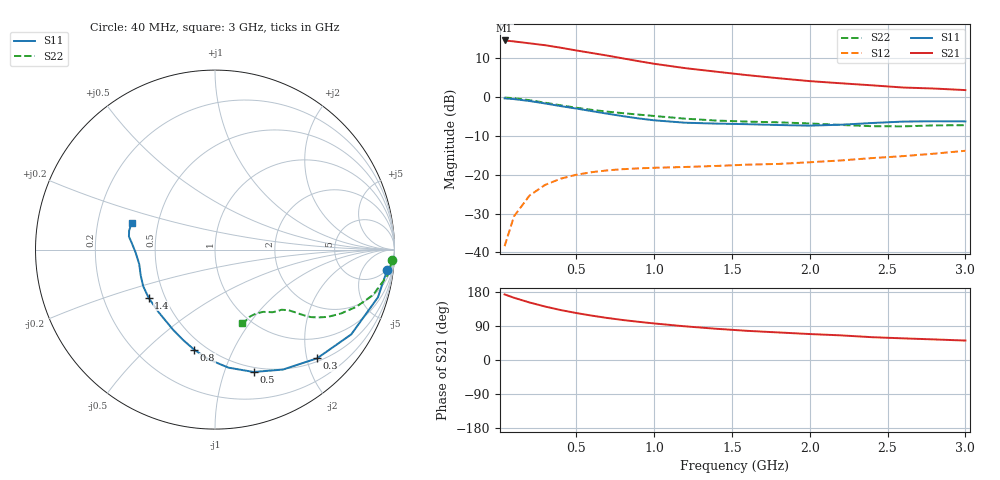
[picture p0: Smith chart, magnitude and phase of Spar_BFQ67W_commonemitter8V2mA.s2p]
! Filename:  BFQ67WG.S2P  Version:  4.0
! NXP part #: BFQ67W  Date: Jun 1994
! Bias condition: Vce=8V, Ic=2mA
#  MHz  S  MA  R  50
! Freq  S11  S21  S12  S22  !GUM [dB]
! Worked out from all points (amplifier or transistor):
!   21 points, 40 MHz to 3 GHz, reference 50 ohm
!   highest |S21| = 14.6 dB at 40 MHz (marker M1)
!   |S21| within 3 dB of that: start of sweep to 564 MHz
!   unconditionally stable (mu >= 1): 1.305 GHz to end of sweep
!   at 300 MHz: K = 0.29, MSG = 18.0 dB, |S12| = -22.6 dB
!   at 1 GHz: K = 0.80, MSG = 13.4 dB, |S12| = -18.2 dB
!   at 3 GHz: K = 1.16, MAG = 5.4 dB, |S12| = -13.8 dB
!   lowest NFmin = 1.30 dB at 1 GHz
!   S11 on the Smith chart (normalised r, x): 40 MHz: 5, -16; 300 MHz: 0.56, -2.19; 500 MHz: 0.45, -1.26; 800 MHz: 0.43, -0.72; 1.4 GHz: 0.41, -0.27; 3 GHz: 0.35, +0.14
40  0.966 -6.7  5.396 173.1  0.012 85.5  0.99 -3.5
100  0.946 -16.3  5.244 164.3  0.029 78.5  0.972 -8.5
200  0.894 -31.9  4.957 151.8  0.054 68.3  0.916 -16.0
300  0.831 -46.8  4.685 141.1  0.074 60.8  0.85 -22.0
400  0.768 -60.5  4.352 131.8  0.089 54.9  0.787 -26.9
500  0.715 -72.5  4.012 124.0  0.1 50.5  0.732 -30.8
600  0.662 -83.5  3.716 117.1  0.108 47.4  0.687 -33.4
700  0.613 -93.2  3.442 110.9  0.114 45.6  0.652 -35.2
800  0.57 -101.7  3.168 105.5  0.118 44.5  0.623 -36.2
900  0.533 -109.7  2.919 100.8  0.121 43.7  0.597 -37.1
1000  0.504 -117.6  2.701 96.5  0.123 43.4  0.573 -37.8
1200  0.469 -132.3  2.372 88.8  0.126 43.9  0.529 -39.6
1400  0.457 -144.1  2.134 82.4  0.13 45.6  0.5 -42.1
1600  0.449 -153.1  1.925 76.9  0.135 47.9  0.485 -45.2
1800  0.438 -160.9  1.757 72.7  0.138 51.5  0.474 -47.4
2000  0.43 -169.3  1.613 68.5  0.145 55.3  0.459 -49.3
2200  0.442 -177.6  1.513 65.0  0.153 59.5  0.439 -52.2
2400  0.465 175.5  1.424 60.2  0.164 62.2  0.423 -57.3
2600  0.485 171.4  1.334 57.1  0.174 64.7  0.421 -63.0
2800  0.49 167.6  1.294 54.3  0.187 68.0  0.433 -66.9
3000  0.488 162.3  1.236 51.3  0.204 70.3  0.436 -69.5
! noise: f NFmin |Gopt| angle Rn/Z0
1000  1.3  0.69  65  0.287
